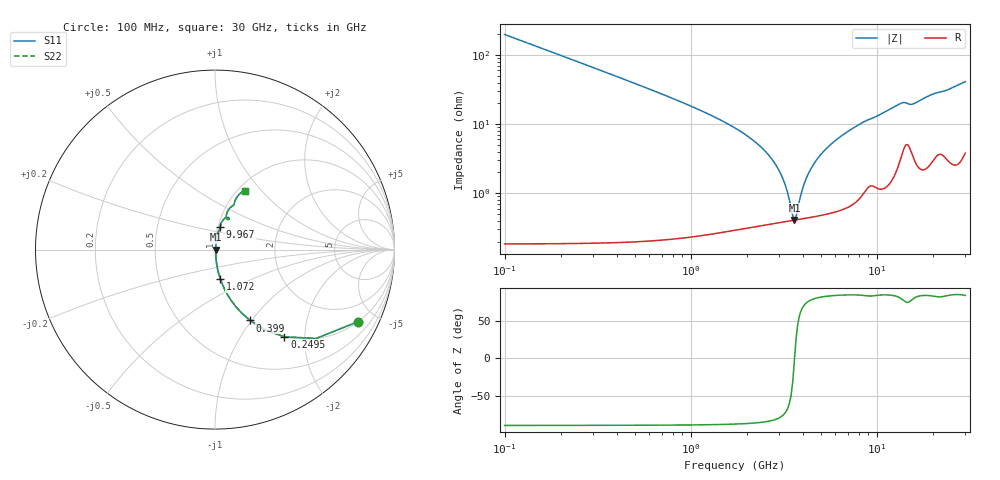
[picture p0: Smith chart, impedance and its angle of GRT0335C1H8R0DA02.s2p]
!Murata Part Number: GRT0335C1H8R0DA02
!These Parameters are Measured in Series Mode Connection
!Data Generated on Jun 19, 2026
!  o--ll--o
!Port1  Port2
!  o------o
!Operation Temp=25[degC], DC Bias Voltage=0[V]
!Freq. Start=100[MHz] Stop=30[GHz] 401[Steps]
# Hz S RI R 50
!Freq.(Hz) S11(Real) S11(Imag) S21(Real) S21(Imag) S12(Real) S12(Imag) S22(Real) S22(Imag)
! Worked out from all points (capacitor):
!   401 points, 100 MHz to 30 GHz, reference 50 ohm
!   read as one part in series: C = 8 pF near 249.5 MHz
!   lowest |Z| = 408 mohm at 3.613 GHz (marker M1)
!   series resonance near 3.621 GHz, so ESL is about 240 pH
!   S11 on the Smith chart (normalised r, x): 100 MHz: 1.00, -3.98; 249.5 MHz: 1.00, -1.59; 399 MHz: 1.00, -0.98; 1.072 GHz: 1.00, -0.34; 9.967 GHz: 1.02, +0.26; 30 GHz: 1.08, +0.82
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1e8  0.7978 -0.4012  0.2022 0.4012  0.2022 0.4012  0.7978 -0.4012
2.495e8  0.3866 -0.4858  0.6134 0.4858  0.6134 0.4858  0.3866 -0.4858
3.99e8  0.196 -0.395  0.804 0.395  0.804 0.395  0.196 -0.395
6.2325e8  0.0889 -0.2812  0.9111 0.2812  0.9111 0.2812  0.0889 -0.2812
1.07175e9  0.0299 -0.1633  0.9701 0.1633  0.9701 0.1633  0.0299 -0.1633
2.791e9  0.00444 -0.0284  0.9956 0.0284  0.9956 0.0284  0.00444 -0.0284
3.09e9  0.00409 -0.0172  0.9959 0.0172  0.9959 0.0172  0.00409 -0.0172
3.46375e9  0.00401 -0.00478  0.996 0.00478  0.996 0.00478  0.00401 -0.00478
3.61325e9  0.00406 -0.00022  0.9959 0.00022  0.9959 0.00022  0.00406 -0.00022
3.76275e9  0.00415 0.00415  0.9958 -0.00415  0.9958 -0.00415  0.00415 0.00415
3.987e9  0.00435 0.0104  0.9956 -0.0104  0.9956 -0.0104  0.00435 0.0104
4.286e9  0.00472 0.0183  0.9953 -0.0183  0.9953 -0.0183  0.00472 0.0183
5.10825e9  0.00624 0.0379  0.9938 -0.0379  0.9938 -0.0379  0.00624 0.0379
5.9305e9  0.00838 0.0555  0.9916 -0.0555  0.9916 -0.0555  0.00838 0.0555
7.05175e9  0.0124 0.0776  0.9876 -0.0776  0.9876 -0.0776  0.0124 0.0776
9.967e9  0.0276 0.1239  0.9724 -0.1239  0.9724 -0.1239  0.0276 0.1239
1.01165e10  0.028 0.1264  0.972 -0.1264  0.972 -0.1264  0.028 0.1264
1.34055e10  0.0638 0.1789  0.9362 -0.1789  0.9362 -0.1789  0.0638 0.1789
1.505e10  0.0733 0.1671  0.9267 -0.1671  0.9267 -0.1671  0.0733 0.1671
2.005825e10  0.0915 0.2393  0.9085 -0.2393  0.9085 -0.2393  0.0915 0.2393
2.50665e10  0.1166 0.2826  0.8834 -0.2826  0.8834 -0.2826  0.1166 0.2826
3e10  0.1658 0.3282  0.8342 -0.3282  0.8342 -0.3282  0.1658 0.3282
